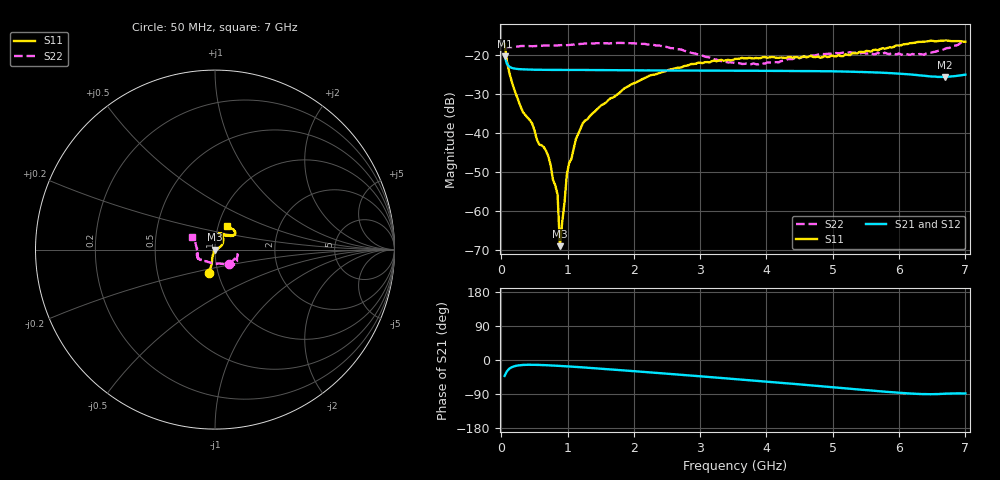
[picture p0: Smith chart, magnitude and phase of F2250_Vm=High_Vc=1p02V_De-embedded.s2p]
! Integrated Device Technology
! Corporate Headquarters
! 6024 Silver Creek Valley Road
! San Jose, CA 95138  USA
! Phone:  1-408-284-8200
! Toll Free:  1-800-223-1366
! Webpage:  http://www.idt.com/
! Timing and RF Division
! 515 Groton Road, Suite 102
! Westford, MA 01886-6024
! Device:  F2250
! Description: Voltage Variable RF Attenuator
! Frequency:  50.0 -  6000.00 MHz
! Package:  3x3 mm Thin QFN Plastic Package: 16 pin
! Ports:  2 RF, 3 DC
!  Pin  1  = GND
!  Pin  2  = NC
!  Pin  3  = RF1  = Port 1
!  Pin  4  = NC
!  Pin  5  = GND
!  Pin  6  = GND
!  Pin  7  = GND
!  Pin  8  = GND
!  Pin  9  = NC
!  Pin 10  = RF2  = Port 2
!  Pin 11  = NC
!  Pin 12  = GND
!  Pin 13  = GND
!  Pin 14  = VCNTRL
!  Pin 15  = VDD
!  Pin 16  = VMODE
! Vcntrl:  1.020 Volts
! Vmode:  +3.300 Volts
! Vdd:  +3.30  Volts
! Current:  1.325 mA
! Data:  The device was measured on a the F2250 evaluation board which has
!  individual transmission lines to the RF pins.  Data was collected
!  using a calibrated network analyzer.  The evaluation board was
!  de-embedded using a TRL calibration technique.
!  The reference plane is the edge of the package pin.
! Misc:  SN 10
!  Action Tracker AT0258
! Date Measured:  2014-11-26
! Date:  2015-10-15  MJV
! Note:
!  Integrated Device Technology supplies this data as a sample of measured
!  data at the package pin for this product.  Your particular data for this
!  product may vary.
!  Data was taken at 25 degrees C.
!  Integrated Device Technology reserves the right to change this data at anytime.
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# GHz S dB R 50
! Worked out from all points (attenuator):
!   201 points, 50 MHz to 7 GHz, reference 50 ohm
!   highest |S21| = -20.41 dB at 50 MHz (marker M1); lowest = -25.7 dB at 6.687 GHz (marker M2)
!   lowest |S11| = -68.9 dB at 884 MHz (marker M3), VSWR 1.00, Z = 50 - j0.0267 ohm
!   |S11| at or under -10 dB: start of sweep to end of sweep
!   |S22| runs from -22.5 to -16.6 dB; largest |S21 - S12| = 0.0003
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0.05  -17.29 -105.2  -20.41 -41.9  -20.41 -41.9  -18.91 -45.5
0.1195  -24.50 -105.6  -23.05 -23.2  -23.06 -23.1  -18.24 -17.0
0.29325  -33.35 -111.7  -23.73 -13.5  -23.72 -13.5  -17.80 -12.6
0.467  -37.65 -125.0  -23.83 -12.6  -23.83 -12.6  -17.86 -13.1
0.57125  -42.93 -132.3  -23.86 -13.0  -23.86 -13.0  -17.78 -15.2
0.71025  -46.02 -130.8  -23.89 -14.0  -23.88 -14.0  -17.66 -17.7
0.77975  -51.97 -150.8  -23.90 -14.6  -23.90 -14.6  -17.69 -18.9
0.84925  -55.77 -160.3  -23.91 -15.3  -23.90 -15.3  -17.64 -20.9
0.884  -68.91 -131.8  -23.90 -15.6  -23.92 -15.6  -17.60 -21.8
0.9535  -57.78 -73.0  -23.92 -16.3  -23.93 -16.3  -17.63 -22.7
0.98825  -50.67 -25.8  -23.94 -16.7  -23.93 -16.7  -17.57 -23.3
1.12725  -41.45 8.7  -23.92 -18.2  -23.91 -18.2  -17.36 -25.3
1.2315  -37.44 13.5  -23.91 -19.5  -23.92 -19.5  -17.19 -27.4
1.857  -28.60 29.4  -23.98 -27.6  -24.00 -27.6  -17.03 -34.4
2.37825  -24.71 40.2  -24.02 -34.5  -24.03 -34.5  -17.65 -40.3
3.525  -21.09 68.7  -24.11 -50.3  -24.12 -50.3  -22.13 -84.0
3.8725  -20.91 75.0  -24.10 -55.1  -24.11 -55.2  -22.49 -108.0
4.7065  -20.60 70.5  -24.20 -67.5  -24.20 -67.5  -20.24 -143.3
5.85325  -18.12 39.0  -24.70 -84.6  -24.70 -84.7  -19.89 -164.2
6.3745  -16.67 39.8  -25.38 -90.1  -25.36 -90.2  -20.02 176.2
6.68725  -16.39 46.9  -25.70 -89.1  -25.69 -89.2  -18.56 158.5
7  -16.69 61.9  -25.11 -88.3  -25.10 -88.5  -16.55 151.2
